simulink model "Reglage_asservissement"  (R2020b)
settings: Solver=FixedStepAuto  StartTime=0.0  StopTime=inf  FixedStep=0.01  RelTol=1e-3  EnableMultiTasking=on
libraries: arduinolib x4, simulink x1, pid_lib x1

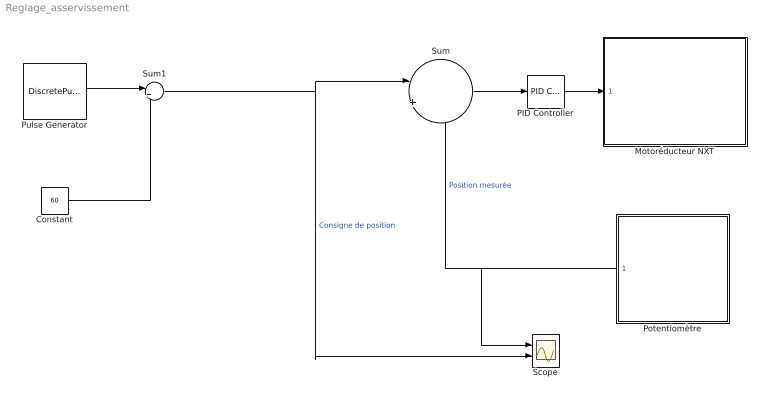
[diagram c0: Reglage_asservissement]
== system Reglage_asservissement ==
  Constant : Constant  Value=60
  Motoréducteur NXT : Subsystem
  PID Controller : pid_lib/PID Controller  Controller=PID  Form=Parallel  TimeDomain=Discrete-time  UseExternalTs=off  SampleTime=-1  IntegratorMethod=Forward Euler  FilterMethod=Forward Euler  ControllerParametersSource=internal  P=0.1  I=0  D=0  UseFilter=on  N=100  TunerSelectOption=Transfer Function Based (PID Tuner App)  InitialConditionSource=internal  InitialConditionForIntegrator=0  InitialConditionForFilter=0  DifferentiatorICPrevScaledInput=0  ExternalReset=none  TrackingMode=off  Kt=1  LimitOutput=off  SatLimitsSource=internal  UpperSaturationLimit=inf  LowerSaturationLimit=-inf  LinearizeAsGain=on  AntiWindupMode=none  Kb=1  POutMin=[]  POutMax=[]  IOutMin=[]  IOutMax=[]  DOutMin=[]  DOutMax=[]  NOutMin=[]  NOutMax=[]  SumOutMin=[]  SumOutMax=[]  SaturationOutMin=[]  SaturationOutMax=[]  PParamMin=[]  PParamMax=[]  IParamMin=[]  IParamMax=[]  DParamMin=[]  DParamMax=[]  NParamMin=[]  NParamMax=[]  KbParamMin=[]  KbParamMax=[]  KtParamMin=[]  KtParamMax=[]  KbOutMin=[]  KbOutMax=[]  KtOutMin=[]  KtOutMax=[]  IntegratorOutMin=[]  IntegratorOutMax=[]  FilterOutMin=[]  FilterOutMax=[]  SumI1OutMin=[]  SumI1OutMax=[]  SumI2OutMin=[]  SumI2OutMax=[]  SumI3OutMin=[]  SumI3OutMax=[]  SumI4OutMin=[]  SumI4OutMax=[]  SumDOutMin=[]  SumDOutMax=[]  DifferentiatorOutMin=[]  DifferentiatorOutMax=[]  FilterDiffOutCoefMin=[]  FilterDiffOutCoefMax=[]  ReciprocalOutMin=[]  ReciprocalOutMax=[]  SumDenOutMin=[]  SumDenOutMax=[]  SumNumOutMin=[]  SumNumOutMax=[]  DivideOutMin=[]  DivideOutMax=[]  UdiffTsProdOutMin=[]  UdiffTsProdOutMax=[]  NTsProdOutMin=[]  NTsProdOutMax=[]  UintegralTsProdOutMin=[]  UintegralTsProdOutMax=[]  UngainTsProdOutMin=[]  UngainTsProdOutMax=[]  IntegratorContinuousStateAttributes=''  IntegratorStateMustResolveToSignalObject=off  IntegratorRTWStateStorageClass=Auto  FilterContinuousStateAttributes=''  FilterStateMustResolveToSignalObject=off  FilterRTWStateStorageClass=Auto  ParallelPVariant=InternalParameters  IdealPVariant=Disabled  IVariant=InternalParameters  DVariant=InternalParameters  IntegratorVariant=Discrete  SatVariant=Disabled  AWVariant=Passthrough  PCopyVariant=Disabled  TRVariant=Disabled  FdbkBlocksVariant=Forward  IdealPFdbkVariant=Disabled  SatFdbkVariant=Disabled  DerivativeFilterVariant=ForwardEulerFilter  NVariant=InternalParameters  NCopyVariant=Disabled  FilterICVariant=InternalICsFilter  IntegratorICVariant=InternalICs  ExternalResetVariant=Disabled  TRSumVariant=Passthrough  SumFdbkVariant=Disabled  SumVariant=Sum_PID  TsampFilterVariant=InternalTs  TsampNgainVariant=Passthrough  TsampIntegralVariant=Passthrough  ExternalSaturationOutDataTypeStr=Inherit: Same as second input
  Potentiomètre : Subsystem
  Pulse Generator : DiscretePulseGenerator  PulseType=Time based  Amplitude=20  Period=4  PulseWidth=50
  Scope : Scope  NumInputPorts=2
  Sum : Sum  Inputs=|+-
  Sum1 : Sum  Inputs=|++
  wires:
  Sum/1 -> PID Controller/1
  PID Controller/1 -> Motoréducteur NXT/1(U)
  Potentiomètre/1(Out1) -> Sum/2, Scope/1  "Position mesurée"
  Sum1/1 -> Sum/1, Scope/2  "Consigne de position"
  Constant/1 -> Sum1/2
  Pulse Generator/1 -> Sum1/1

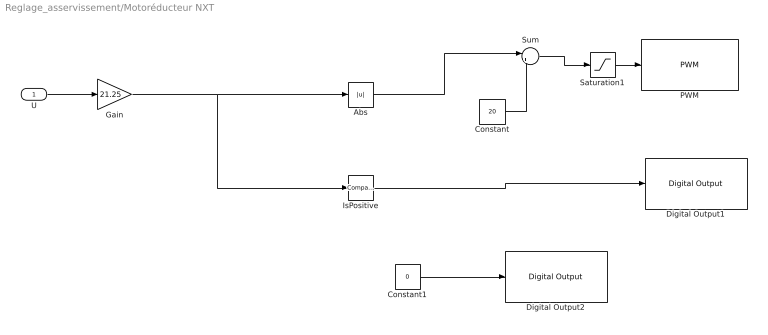
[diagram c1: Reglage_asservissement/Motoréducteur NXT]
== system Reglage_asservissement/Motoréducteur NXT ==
  U : Inport
  Abs : Abs
  Constant : Constant  Value=20
  Constant1 : Constant  Value=0
  Digital Output1 : arduinolib/Digital Output  pinNumber=12  Direction=output  blockPlatform=arduino
  Digital Output2 : arduinolib/Digital Output  pinNumber=9  Direction=output  blockPlatform=arduino
  Gain : Gain  Gain=21.25
  IsPositive : simulink/Logic and Bit Operations/Compare To Zero  relop=>  OutDataTypeStr=boolean
  PWM : arduinolib/PWM  pinNumber=3  frequencyType=Default  desiredFrequency=490.2  achievableFrequency=490.2
  Saturation1 : Saturate  UpperLimit=255  LowerLimit=0
  Sum : Sum  Inputs=|++
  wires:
  U/1 -> Gain/1
  Constant1/1 -> Digital Output2/1
  Sum/1 -> Saturation1/1
  Saturation1/1 -> PWM/1
  Constant/1 -> Sum/2
  IsPositive/1 -> Digital Output1/1
  Abs/1 -> Sum/1
  Gain/1 -> Abs/1, IsPositive/1

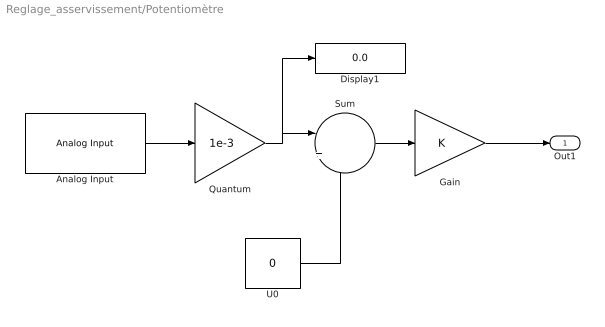
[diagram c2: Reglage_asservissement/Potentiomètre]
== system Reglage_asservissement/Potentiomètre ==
  Analog Input : arduinolib/Analog Input  pinNumber=0  ReadResultsOnly=off  ConversionTriggerSource=Software  ExternalTriggerType=uint32(0)  OutputDataType=uint16  EnableConversionCompleteNotify=off  EnableOuputStatus=off  SampleTime=0.01  blockPlatform=arduino
  Display1 : Display
  Gain : Gain
  Quantum : Gain  Gain=1e-3
  Sum : Sum  Inputs=|+-
  U0 : Constant  Value=0
  Out1 : Outport  VectorParamsAs1DForOutWhenUnconnected=off
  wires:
  Gain/1 -> Out1/1
  Analog Input/1 -> Quantum/1
  Quantum/1 -> Display1/1, Sum/1
  U0/1 -> Sum/2
  Sum/1 -> Gain/1
